| TEXAS INSTRUMENTS INCORPORATED
| Standard Linear and Logic Group
| IBIS Model of SN74AHC540
| OCTAL BUFFERS/DRIVERS WITH 3-STATE OUTPUTS
| This file contains package information for the following:
|  SSOP 20-pin (DB) package as [Component] AHC540_DB
|  TVSOP 20-pin (DGV) package as [Component] AHC540_DGV
|  SOIC 20-pin (DW) package as [Component] AHC540_DW
|  PDIP 20-pin (N) package as [Component] AHC540_N
|  SOP 20-pin (NS) package as [Component] AHC540_NS
|  TSSOP 20-pin (PW) package as [Component] AHC540_PW
| This device can be powered at the following Vccs:
|  2.2 volt Vcc
|  3.3 volt Vcc
|  5 volt Vcc
| This file provides unique models under the [Model Selector] for each Vcc.
| For operation at a specific Vcc, select the appropriate model after each
| [Model Selector] keyword.
[IBIS Ver]   3.2
[Comment char]  |_char
[File Name]   sn74ahc540.ibs
[File Rev]   1.1 | a_die
[Date]   November 14, 2002
[Source]   Data created from TI-SPICE simulations at TI-SLL.
[Notes]   The following is an IBIS list for the AHC540.
   Please contact sllibis@ti.com with questions and
   comments concerning SLL IBIS models.
   -This IBIS model is created from a BA (back annotated
   netlist)
   -Power clamp data has been deleted from the input model
[Disclaimer] Property of Texas Instruments Incorporated.  Unauthorized
   reproduction and/or distribution is strictly prohibited.
   This product is protected under copyright law.
   Created  2002, (C) Copyright  2002, Texas Instruments
   Incorporated, All Rights Reserved
   UNLESS THERE IS A SIGNED, WRITTEN AGREEMENT TO THE
   CONTRARY, TEXAS INSTRUMENTS (TI) IS PROVIDING THE IBIS
   MODELS  AND WITHOUT ANY WARRANTY, EXPRESSED OR
   IMPLIED.  TI assumes no liability for:
   1) the accuracy of the IBIS models provided to your
   company;
   2) the proper functioning of these IBIS Models in your
   design or for any resulting applications; or
   3) infringement of patents, copyrights or intellectual
   property rights resulting from your use of these IBIS
   models.
   TI provides IBIS Models as a service to our customers.
   You and your company shall not distribute, sell or give
   these models to anyone else without prior written
   permission from TI.
   TI reserves the right to make changes to our products or
   to discontinue any semiconductor product or service
   without notice, and advises our customers to obtain the
   latest version of relevant information to verify, before
   placing orders, that the information being relied on is
   current.
   Please be aware that your receipt and use of the IBIS
   information provided shall serve as acceptance of these
   terms and conditions.  If you do not accept these terms,
   you should return or destroy the IBIS models and any
   other accompanying information immediately.
| Component AHC540_DB 20-pin SSOP
[Component]   AHC540_DB
[Manufacturer]   Texas Instruments, Inc.
[Package]
|   typ   min   max
R_pkg   4.000e-02   3.500e-02   5.100e-02
L_pkg   3.495e-09   3.035e-09   4.314e-09
C_pkg   4.200e-13   3.460e-13   5.020e-13
[Pin]   signal_name   model_name   R_pin   L_pin   C_pin
1   NOE1   AHC540_NOE   4.900e-02   4.310e-09   5.020e-13
2   A1   AHC540_IN   4.800e-02   3.903e-09   4.870e-13
3   A2   AHC540_IN   3.500e-02   3.189e-09   3.960e-13
4   A3   AHC540_IN   3.500e-02   3.036e-09   3.470e-13
5   A4   AHC540_IN   3.500e-02   3.035e-09   3.670e-13
6   A5   AHC540_IN   3.500e-02   3.035e-09   3.670e-13
7   A6   AHC540_IN   3.500e-02   3.036e-09   3.470e-13
8   A7   AHC540_IN   3.500e-02   3.189e-09   3.970e-13
9   A8   AHC540_IN   4.700e-02   3.899e-09   4.880e-13
10   GND   GND   5.100e-02   4.314e-09   5.000e-13
11   Y8   AHC540_OUT   5.100e-02   4.314e-09   5.000e-13
12   Y7   AHC540_OUT   4.700e-02   3.899e-09   4.880e-13
13   Y6   AHC540_OUT   3.500e-02   3.189e-09   3.970e-13
14   Y5   AHC540_OUT   3.500e-02   3.036e-09   3.460e-13
15   Y4   AHC540_OUT   3.500e-02   3.035e-09   3.670e-13
16   Y3   AHC540_OUT   3.500e-02   3.035e-09   3.670e-13
17   Y2   AHC540_OUT   3.500e-02   3.036e-09   3.460e-13
18   Y1   AHC540_OUT   3.500e-02   3.189e-09   3.970e-13
19   NOE2   AHC540_NOE   4.700e-02   3.899e-09   4.880e-13
20   VCC   POWER   5.100e-02   4.314e-09   5.020e-13
| Component AHC540_DGV 20-pin TVSOP
[Component]   AHC540_DGV
[Manufacturer]   Texas Instruments, Inc.
[Package]
|   typ   min   max
R_pkg   4.400e-02   3.800e-02   4.800e-02
L_pkg   2.561e-09   2.236e-09   2.961e-09
C_pkg   3.420e-13   2.640e-13   4.460e-13
[Pin]   signal_name   model_name   R_pin   L_pin   C_pin
1   NOE1   AHC540_NOE   4.400e-02   2.935e-09   4.170e-13
2   A1   AHC540_IN   4.200e-02   2.869e-09   4.460e-13
3   A2   AHC540_IN   4.300e-02   2.399e-09   3.160e-13
4   A3   AHC540_IN   4.400e-02   2.236e-09   2.650e-13
5   A4   AHC540_IN   4.600e-02   2.278e-09   2.640e-13
6   A5   AHC540_IN   4.500e-02   2.274e-09   2.640e-13
7   A6   AHC540_IN   4.400e-02   2.285e-09   2.690e-13
8   A7   AHC540_IN   4.300e-02   2.452e-09   3.200e-13
9   A8   AHC540_IN   4.400e-02   2.900e-09   4.460e-13
10   GND   GND   4.400e-02   2.961e-09   4.180e-13
11   Y8   AHC540_OUT   4.500e-02   2.954e-09   4.180e-13
12   Y7   AHC540_OUT   4.200e-02   2.847e-09   4.430e-13
13   Y6   AHC540_OUT   4.500e-02   2.453e-09   3.190e-13
14   Y5   AHC540_OUT   4.500e-02   2.297e-09   2.690e-13
15   Y4   AHC540_OUT   4.800e-02   2.334e-09   2.680e-13
16   Y3   AHC540_OUT   4.800e-02   2.335e-09   2.670e-13
17   Y2   AHC540_OUT   4.600e-02   2.299e-09   2.680e-13
18   Y1   AHC540_OUT   4.600e-02   2.457e-09   3.200e-13
19   NOE2   AHC540_NOE   4.300e-02   2.848e-09   4.410e-13
20   VCC   POWER   3.800e-02   2.812e-09   4.080e-13
| Component AHC540_DW 20-pin SOIC
[Component]   AHC540_DW
[Manufacturer]   Texas Instruments, Inc.
[Package]
|   typ   min   max
R_pkg   3.800e-02   3.300e-02   4.500e-02
L_pkg   5.012e-09   4.110e-09   6.349e-09
C_pkg   7.170e-13   5.300e-13   8.680e-13
[Pin]   signal_name   model_name   R_pin   L_pin   C_pin
1   NOE1   AHC540_NOE   4.200e-02   6.336e-09   8.650e-13
2   A1   AHC540_IN   4.300e-02   5.542e-09   8.670e-13
3   A2   AHC540_IN   3.400e-02   4.714e-09   7.320e-13
4   A3   AHC540_IN   3.400e-02   4.377e-09   5.910e-13
5   A4   AHC540_IN   3.600e-02   4.130e-09   5.330e-13
6   A5   AHC540_IN   3.500e-02   4.111e-09   5.300e-13
7   A6   AHC540_IN   3.400e-02   4.284e-09   5.830e-13
8   A7   AHC540_IN   3.400e-02   4.634e-09   7.260e-13
9   A8   AHC540_IN   4.000e-02   5.518e-09   8.650e-13
10   GND   GND   4.300e-02   6.349e-09   8.660e-13
11   Y8   AHC540_OUT   4.100e-02   6.281e-09   8.610e-13
12   Y7   AHC540_OUT   4.500e-02   5.561e-09   8.680e-13
13   Y6   AHC540_OUT   3.300e-02   4.778e-09   7.420e-13
14   Y5   AHC540_OUT   3.500e-02   4.414e-09   5.960e-13
15   Y4   AHC540_OUT   3.500e-02   4.110e-09   5.330e-13
16   Y3   AHC540_OUT   3.600e-02   4.130e-09   5.330e-13
17   Y2   AHC540_OUT   3.400e-02   4.377e-09   5.910e-13
18   Y1   AHC540_OUT   3.400e-02   4.714e-09   7.310e-13
19   NOE2   AHC540_NOE   4.300e-02   5.569e-09   8.680e-13
20   VCC   POWER   4.200e-02   6.308e-09   8.640e-13
| Component AHC540_N 20-pin PDIP
[Component]   AHC540_N
[Manufacturer]   Texas Instruments, Inc.
[Package]
|   typ   min   max
R_pkg   4.300e-02   3.800e-02   5.000e-02
L_pkg   7.384e-09   4.680e-09   1.032e-08
C_pkg   5.100e-13   2.310e-13   8.210e-13
[Pin]   signal_name   model_name   R_pin   L_pin   C_pin
1   NOE1   AHC540_NOE   4.200e-02   9.427e-09   8.100e-13
2   A1   AHC540_IN   4.600e-02   8.544e-09   4.560e-13
3   A2   AHC540_IN   4.800e-02   7.163e-09   4.350e-13
4   A3   AHC540_IN   4.000e-02   4.825e-09   2.610e-13
5   A4   AHC540_IN   4.000e-02   5.284e-09   6.480e-13
6   A5   AHC540_IN   4.000e-02   4.686e-09   2.320e-13
7   A6   AHC540_IN   4.000e-02   6.359e-09   4.890e-13
8   A7   AHC540_IN   3.800e-02   7.982e-09   4.750e-13
9   A8   AHC540_IN   4.300e-02   9.403e-09   4.750e-13
10   GND   GND   5.000e-02   1.032e-08   8.050e-13
11   Y8   AHC540_OUT   5.000e-02   1.028e-08   8.100e-13
12   Y7   AHC540_OUT   4.300e-02   9.383e-09   4.770e-13
13   Y6   AHC540_OUT   3.800e-02   7.978e-09   4.760e-13
14   Y5   AHC540_OUT   4.000e-02   6.302e-09   4.920e-13
15   Y4   AHC540_OUT   4.000e-02   4.680e-09   2.310e-13
16   Y3   AHC540_OUT   4.000e-02   5.284e-09   6.480e-13
17   Y2   AHC540_OUT   4.000e-02   4.822e-09   2.610e-13
18   Y1   AHC540_OUT   4.700e-02   7.118e-09   4.390e-13
19   NOE2   AHC540_NOE   4.600e-02   8.492e-09   4.610e-13
20   VCC   POWER   4.300e-02   9.348e-09   8.210e-13
| Component AHC540_NS 20-pin SOP
[Component]   AHC540_NS
[Manufacturer]   Texas Instruments, Inc.
[Package]
|   typ   min   max
R_pkg   4.400e-02   2.900e-02   5.800e-02
L_pkg   3.666e-09   2.317e-09   5.115e-09
C_pkg   5.480e-13   3.160e-13   7.250e-13
[Pin]   signal_name   model_name   R_pin   L_pin   C_pin
1   NOE1   AHC540_NOE   5.800e-02   5.115e-09   7.250e-13
2   A1   AHC540_IN   5.300e-02   4.591e-09   7.240e-13
3   A2   AHC540_IN   4.900e-02   3.754e-09   5.720e-13
4   A3   AHC540_IN   2.900e-02   2.549e-09   3.880e-13
5   A4   AHC540_IN   3.100e-02   2.317e-09   3.160e-13
6   A5   AHC540_IN   3.100e-02   2.317e-09   3.160e-13
7   A6   AHC540_IN   2.900e-02   2.556e-09   3.990e-13
8   A7   AHC540_IN   4.900e-02   3.754e-09   5.790e-13
9   A8   AHC540_IN   5.300e-02   4.591e-09   7.240e-13
10   GND   GND   5.800e-02   5.115e-09   7.250e-13
11   Y8   AHC540_OUT   5.800e-02   5.115e-09   7.250e-13
12   Y7   AHC540_OUT   5.300e-02   4.591e-09   7.240e-13
13   Y6   AHC540_OUT   4.900e-02   3.754e-09   5.790e-13
14   Y5   AHC540_OUT   2.900e-02   2.557e-09   3.990e-13
15   Y4   AHC540_OUT   3.100e-02   2.317e-09   3.160e-13
16   Y3   AHC540_OUT   3.100e-02   2.317e-09   3.160e-13
17   Y2   AHC540_OUT   2.900e-02   2.557e-09   3.990e-13
18   Y1   AHC540_OUT   4.900e-02   3.754e-09   5.790e-13
19   NOE2   AHC540_NOE   5.300e-02   4.591e-09   7.240e-13
20   VCC   POWER   5.800e-02   5.115e-09   7.250e-13
| Component AHC540_PW 20-pin TSSOP
[Component]   AHC540_PW
[Manufacturer]   Texas Instruments, Inc.
[Package]
|   typ   min   max
R_pkg   5.000e-02   4.200e-02   6.000e-02
L_pkg   2.802e-09   2.248e-09   3.553e-09
C_pkg   3.170e-13   2.020e-13   4.430e-13
[Pin]   signal_name   model_name   R_pin   L_pin   C_pin
1   NOE1   AHC540_NOE   5.500e-02   3.461e-09   4.400e-13
2   A1   AHC540_IN   5.500e-02   3.150e-09   4.010e-13
3   A2   AHC540_IN   4.200e-02   2.619e-09   3.020e-13
4   A3   AHC540_IN   4.500e-02   2.273e-09   2.020e-13
5   A4   AHC540_IN   4.500e-02   2.248e-09   2.240e-13
6   A5   AHC540_IN   4.500e-02   2.273e-09   2.260e-13
7   A6   AHC540_IN   4.400e-02   2.323e-09   2.050e-13
8   A7   AHC540_IN   4.600e-02   2.704e-09   3.070e-13
9   A8   AHC540_IN   6.000e-02   3.265e-09   4.110e-13
10   GND   GND   5.700e-02   3.506e-09   4.360e-13
11   Y8   AHC540_OUT   5.800e-02   3.553e-09   4.370e-13
12   Y7   AHC540_OUT   5.800e-02   3.193e-09   4.050e-13
13   Y6   AHC540_OUT   4.200e-02   2.704e-09   3.110e-13
14   Y5   AHC540_OUT   4.600e-02   2.392e-09   2.100e-13
15   Y4   AHC540_OUT   4.700e-02   2.334e-09   2.290e-13
16   Y3   AHC540_OUT   4.700e-02   2.300e-09   2.270e-13
17   Y2   AHC540_OUT   4.700e-02   2.349e-09   2.070e-13
18   Y1   AHC540_OUT   4.500e-02   2.677e-09   3.060e-13
19   NOE2   AHC540_NOE   6.000e-02   3.235e-09   4.060e-13
20   VCC   POWER   5.600e-02   3.487e-09   4.430e-13
| Model AHC540_NOE
[Model Selector]   AHC540_NOE
AHC540_NOE_22   2.2 volt Vcc
AHC540_NOE_33   3.3 volt Vcc
AHC540_NOE_50   5 volt Vcc
| Model AHC540_IN
[Model Selector]   AHC540_IN
AHC540_IN_22   2.2 volt Vcc
AHC540_IN_33   3.3 volt Vcc
AHC540_IN_50   5 volt Vcc
| Model AHC540_OUT
[Model Selector]   AHC540_OUT
AHC540_OUT_22   2.2 volt Vcc
AHC540_OUT_33   3.3 volt Vcc
AHC540_OUT_50   5 volt Vcc
| Models and submodels in the file (9): AHC540_NOE_22 (Input), AHC540_NOE_33 (Input), AHC540_NOE_50 (Input), AHC540_IN_22 (Input), AHC540_IN_33 (Input), AHC540_IN_50 (Input), AHC540_OUT_22 (3-state), AHC540_OUT_33 (3-state), AHC540_OUT_50 (3-state)
